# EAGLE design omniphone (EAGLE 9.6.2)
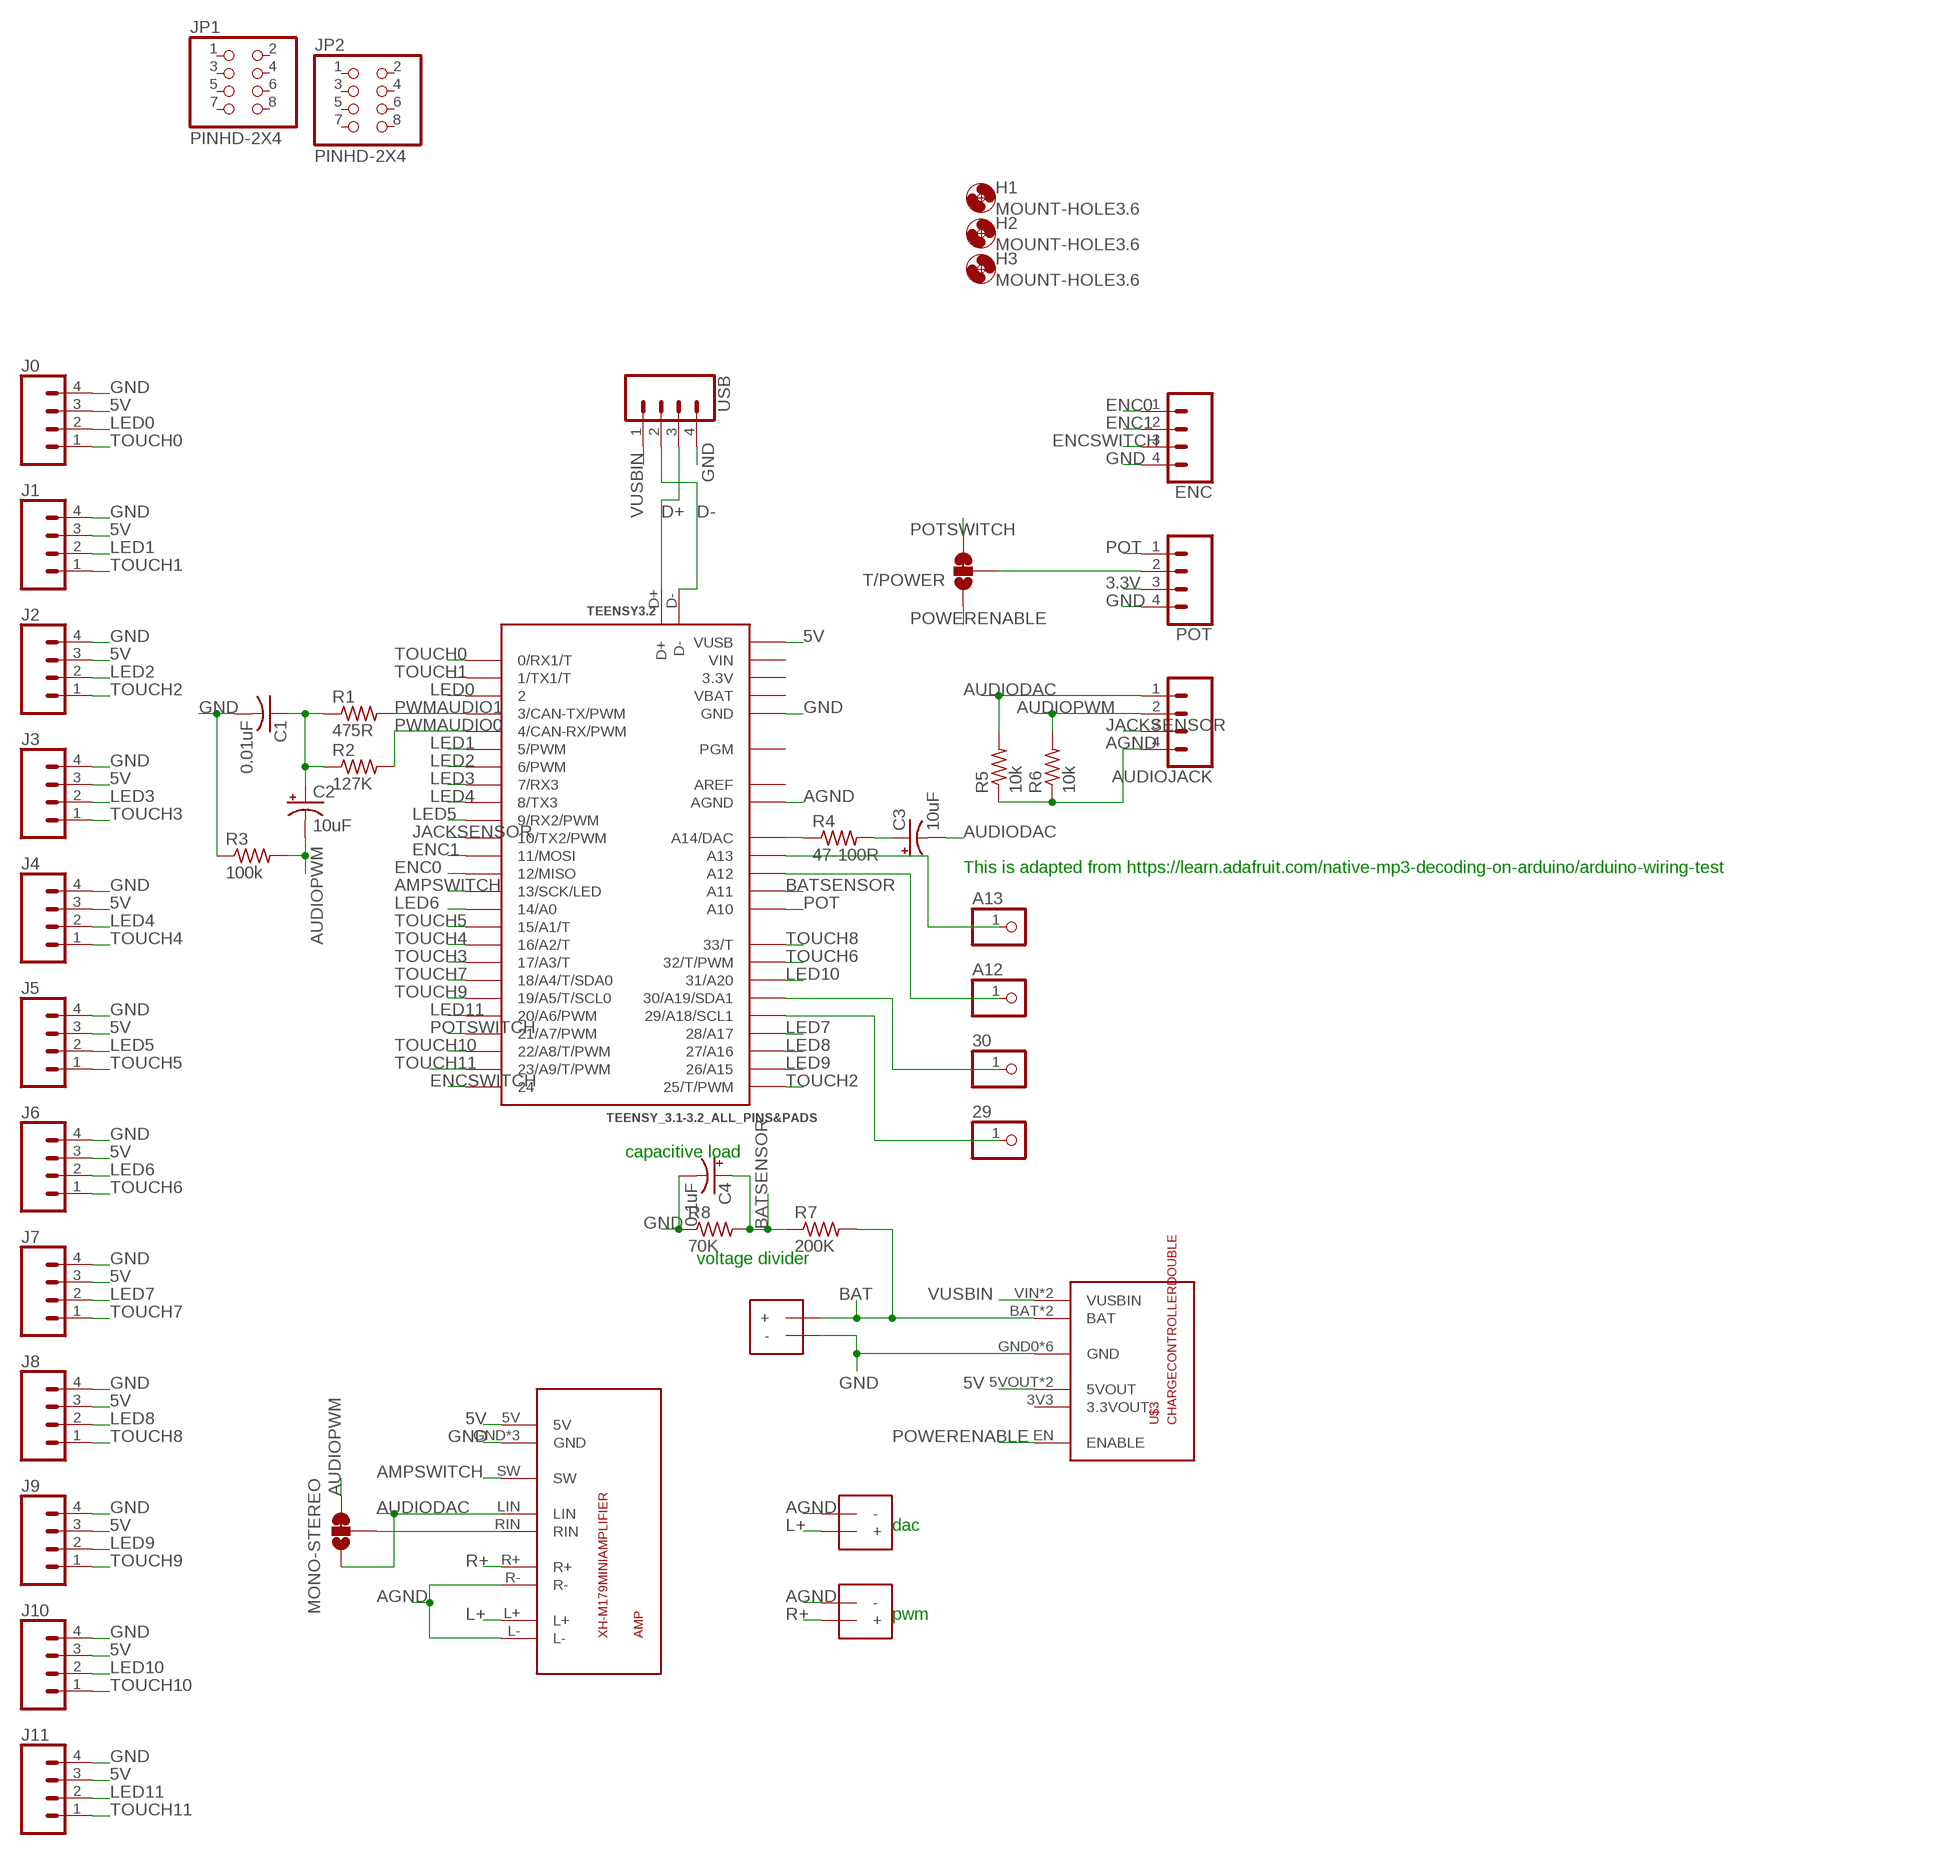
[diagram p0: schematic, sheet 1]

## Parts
29  PINHD-1X1  [1X01]
30  PINHD-1X1  [1X01]
A12  PINHD-1X1  [1X01]
A13  PINHD-1X1  [1X01]
AMP  XH-M179MINIAMPLIFIER  [XH-M179AMP]
AUDIOJACK  CONN_04POLAR_LOCK  [MOLEX-1X4_LOCK]
BATTERY  SPEAKERTERMINAL-3.5MM  [1X2-3.5MM]
C1  0.01uF  C-US025-024X044  [C025-024X044]
C2  10uF  CPOL-USE2-4  [E2-4]
C3  10uF  CPOL-USE2-4  [E2-4]
C4  0.1uF  CPOL-USE2-4  [E2-4]
ENC  CONN_04POLAR_LOCK  [MOLEX-1X4_LOCK]
H1  MOUNT-HOLE3.6  [3,6]
H2  MOUNT-HOLE3.6  [3,6]
H3  MOUNT-HOLE3.6  [3,6]
J0  CONN_04POLAR_LOCK  [MOLEX-1X4_LOCK]
J1  CONN_04POLAR_LOCK  [MOLEX-1X4_LOCK]
J2  CONN_04POLAR_LOCK  [MOLEX-1X4_LOCK]
J3  CONN_04POLAR_LOCK  [MOLEX-1X4_LOCK]
J4  CONN_04POLAR_LOCK  [MOLEX-1X4_LOCK]
J5  CONN_04POLAR_LOCK  [MOLEX-1X4_LOCK]
J6  CONN_04POLAR_LOCK  [MOLEX-1X4_LOCK]
J7  CONN_04POLAR_LOCK  [MOLEX-1X4_LOCK]
J8  CONN_04POLAR_LOCK  [MOLEX-1X4_LOCK]
J9  CONN_04POLAR_LOCK  [MOLEX-1X4_LOCK]
J10  CONN_04POLAR_LOCK  [MOLEX-1X4_LOCK]
J11  CONN_04POLAR_LOCK  [MOLEX-1X4_LOCK]
JP1  PINHD-2X4  [2X04]
JP2  PINHD-2X4  [2X04]
MONO-STEREO  JUMPER-SMT_3_1-NC_TRACE_SILK  [SMT-JUMPER_3_1-NC_TRACE_SILK]
POT  CONN_04POLAR_LOCK  [MOLEX-1X4_LOCK]
R1  475R  R-US_0204/2V  [0204V]
R2  127K  R-US_0204/2V  [0204V]
R3  100k  R-US_0204/2V  [0204V]
R4  47-100R  R-US_0204/2V  [0204V]
R5  10k  R-US_0204/2V  [0204V]
R6  10k  R-US_0204/2V  [0204V]
R7  200K  R-US_0204/2V  [0204V]
R8  70K  R-US_0204/2V  [0204V]
SPEAKERDAC  SPEAKERTERMINAL-3.5MM  [1X2-3.5MM]
SPEAKERPWM  SPEAKERTERMINAL-3.5MM  [1X2-3.5MM]
T/POWER  JUMPER-SMT_3_1-NC_TRACE_SILK  [SMT-JUMPER_3_1-NC_TRACE_SILK]
TEENSY3.2  TEENSY_3.1-3.2_ALL_PINS&PADS  [TEENSY_3.0-3.2_ALL_PINS_&_PADS]
U$3  CHARGECONTROLLERDOUBLE  [CHARGECONTROLLERDOUBLE]
USB  CONN_04POLAR_LOCK  [MOLEX-1X4_LOCK]

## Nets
3.3V: POT.3
5V: AMP.5V J0.3 J1.3 J2.3 J3.3 J4.3 J5.3 J6.3 J7.3 J8.3 J9.3 J10.3 J11.3 TEENSY3.2.VUSB TEENSY3.2.VUSB1(VUSB) U$3.5VOUT U$3.5VOUT1(5VOUT)
AGND: AMP.L- AMP.R- AUDIOJACK.4 R5.1 R6.1 SPEAKERDAC.- SPEAKERPWM.- TEENSY3.2.AGND
AMPSWITCH: AMP.SW TEENSY3.2.13(13/SCK/LED)
AUDIODAC: AMP.LIN AUDIOJACK.1 C3.- MONO-STEREO.1 R5.2
AUDIOPWM: AUDIOJACK.2 C2.- MONO-STEREO.3 R3.2 R6.2
BAT: BATTERY.+ R7.2 U$3.BAT U$3.BAT1(BAT)
BATSENSOR: C4.+ R7.1 R8.2 TEENSY3.2.A11
D+: TEENSY3.2.D+ USB.3
D-: TEENSY3.2.D- USB.2
ENC0: ENC.1 TEENSY3.2.12(12/MISO)
ENC1: ENC.2 TEENSY3.2.11(11/MOSI)
ENCSWITCH: ENC.3 TEENSY3.2.24
GND: AMP.GND AMP.GND1(GND) AMP.GND2(GND) BATTERY.- C1.2 C4.- ENC.4 J0.4 J1.4 J2.4 J3.4 J4.4 J5.4 J6.4 J7.4 J8.4 J9.4 J10.4 J11.4 POT.4 R3.1 R8.1 TEENSY3.2.GND TEENSY3.2.GND1(GND) TEENSY3.2.GND2(GND) TEENSY3.2.GND3(GND) U$3.GND0(GND) U$3.GND1(GND) U$3.GND2(GND) U$3.GND3(GND) U$3.GND4(GND) U$3.GND5(GND) USB.4
JACKSENSOR: AUDIOJACK.3 TEENSY3.2.10(10/TX2/PWM)
L+: AMP.L+ SPEAKERDAC.+
LED0: J0.2 TEENSY3.2.2
LED1: J1.2 TEENSY3.2.5(5/PWM)
LED2: J2.2 TEENSY3.2.6(6/PWM)
LED3: J3.2 TEENSY3.2.7(7/RX3)
LED4: J4.2 TEENSY3.2.8(8/TX3)
LED5: J5.2 TEENSY3.2.9(9/RX2/PWM)
LED6: J6.2 TEENSY3.2.14/A0
LED7: J7.2 TEENSY3.2.28(28/A17)
LED8: J8.2 TEENSY3.2.27(27/A16)
LED9: J9.2 TEENSY3.2.26(26/A15)
LED10: J10.2 TEENSY3.2.31(31/A20)
LED11: J11.2 TEENSY3.2.20/A6(20/A6/PWM)
N$1: C1.1 C2.+ R1.1 R2.1
N$2: A13.1 TEENSY3.2.A13
N$3: A12.1 TEENSY3.2.A12
N$4: POT.2 T/POWER.2
N$5: R4.1 TEENSY3.2.RESET/DAC(A14/DAC)
N$6: 30.1 TEENSY3.2.30(30/A19/SDA1)
N$7: C3.+ R4.2
N$8: 29.1 TEENSY3.2.29(29/A18/SCL1)
POT: POT.1 TEENSY3.2.A10
POTSWITCH: T/POWER.3 TEENSY3.2.21/A7(21/A7/PWM)
POWERENABLE: T/POWER.1 U$3.EN(ENABLE)
PWMAUDIO0: R2.2 TEENSY3.2.4(4/CAN-RX/PWM)
PWMAUDIO1: R1.2 TEENSY3.2.3(3/CAN-TX/PWM)
R+: AMP.R+ SPEAKERPWM.+
RIN: AMP.RIN MONO-STEREO.2
TOUCH0: J0.1 TEENSY3.2.0(0/RX1/T)
TOUCH1: J1.1 TEENSY3.2.1(1/TX1/T)
TOUCH2: J2.1 TEENSY3.2.25(25/T/PWM)
TOUCH3: J3.1 TEENSY3.2.17/A3(17/A3/T)
TOUCH4: J4.1 TEENSY3.2.16/A2(16/A2/T)
TOUCH5: J5.1 TEENSY3.2.15/A1(15/A1/T)
TOUCH6: J6.1 TEENSY3.2.32(32/T/PWM)
TOUCH7: J7.1 TEENSY3.2.18/A4(18/A4/T/SDA0)
TOUCH8: J8.1 TEENSY3.2.33(33/T)
TOUCH9: J9.1 TEENSY3.2.19/A5(19/A5/T/SCL0)
TOUCH10: J10.1 TEENSY3.2.22/A8(22/A8/T/PWM)
TOUCH11: J11.1 TEENSY3.2.23/A9(23/A9/T/PWM)
VUSBIN: U$3.VIN1(VUSBIN) U$3.VIN(VUSBIN) USB.1
Unconnected: JP1.1 JP1.2 JP1.3 JP1.4 JP1.5 JP1.6 JP1.7 JP1.8 JP2.1 JP2.2 JP2.3 JP2.4 JP2.5 JP2.6 JP2.7 JP2.8 TEENSY3.2.PGM U$3.3V3(3.3VOUT)

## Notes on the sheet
- This is adapted from https://learn.adafruit.com/native-mp3-decoding-on-arduino/arduino-wiring-test
- capacitive load
- voltage divider
- dac
- pwm

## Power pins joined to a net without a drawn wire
3.3V: TEENSY3.2.3.3V TEENSY3.2.3.3V1(3.3V) TEENSY3.2.3.3V2(3.3V)
AREF: TEENSY3.2.AREF
VBAT: TEENSY3.2.VBAT
VIN: TEENSY3.2.VIN

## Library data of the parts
29 30 A12 A13 = adafruit:PINHD-1X1: Pin header 1x1 for 0.1" spacing
AMP = ArvidLibrary:XH-M179MINIAMPLIFIER
AUDIOJACK ENC J0 J1-J11 POT USB = SparkFun-Connectors:CONN_04: Multi connection point. Often used as Generic Header-pin footprint for 0.1 inch spaced/style header connections On any of the 0.1 inch spaced packages, you can populate with these: Break Away Headers - Straight (PRT-00116) Break Away Male Headers - Right Angle (PRT-00553) Female Headers (PRT-00115)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; PROD_ID: CONN-08186; SF_ID: PRT-08231
BATTERY SPEAKERDAC SPEAKERPWM = ArvidLibrary:SPEAKERTERMINAL: 3.5mm Terminal block
C1 = adafruit:C-US: CAPACITOR, American symbol
C2-C4 = adafruit:CPOL-US: POLARIZED CAPACITOR, American symbol
H1-H3 = holes:MOUNT-HOLE: MOUNTING HOLE with drill center marker
JP1 JP2 = Connector:PINHD-2X4: PIN HEADER; CATEGORY: CONNECTOR; SUB-CATEGORY: PIN-HEADER
MONO-STEREO T/POWER = SparkFun-Jumpers:JUMPER-SMT_3_1-NC_TRACE: Normally closed trace jumper (1 of 2 connections) This jumper has a trace between two pads so it's normally closed (NC). The other connection is normally open (NO). Use a razor knife to open the connection. For best results follow the IPC guidelines for cutting traces: Cutout at least 0.063 mm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
R1-R8 = adafruit:R-US_: RESISTOR, American symbol
TEENSY3.2 = ArvidLibrary:TEENSY_3.1-3.2_ALL_PINS&PADS: Footprint for Teensy 3.1 or 3.2 board using all pads and all through-holes. Pads need a 2x7 0.1" SMD header. Arvid edit: added USB data and flipped inner pins for easier assembly
U$3 = ArvidLibrary:CHARGECONTROLLERDOUBLE

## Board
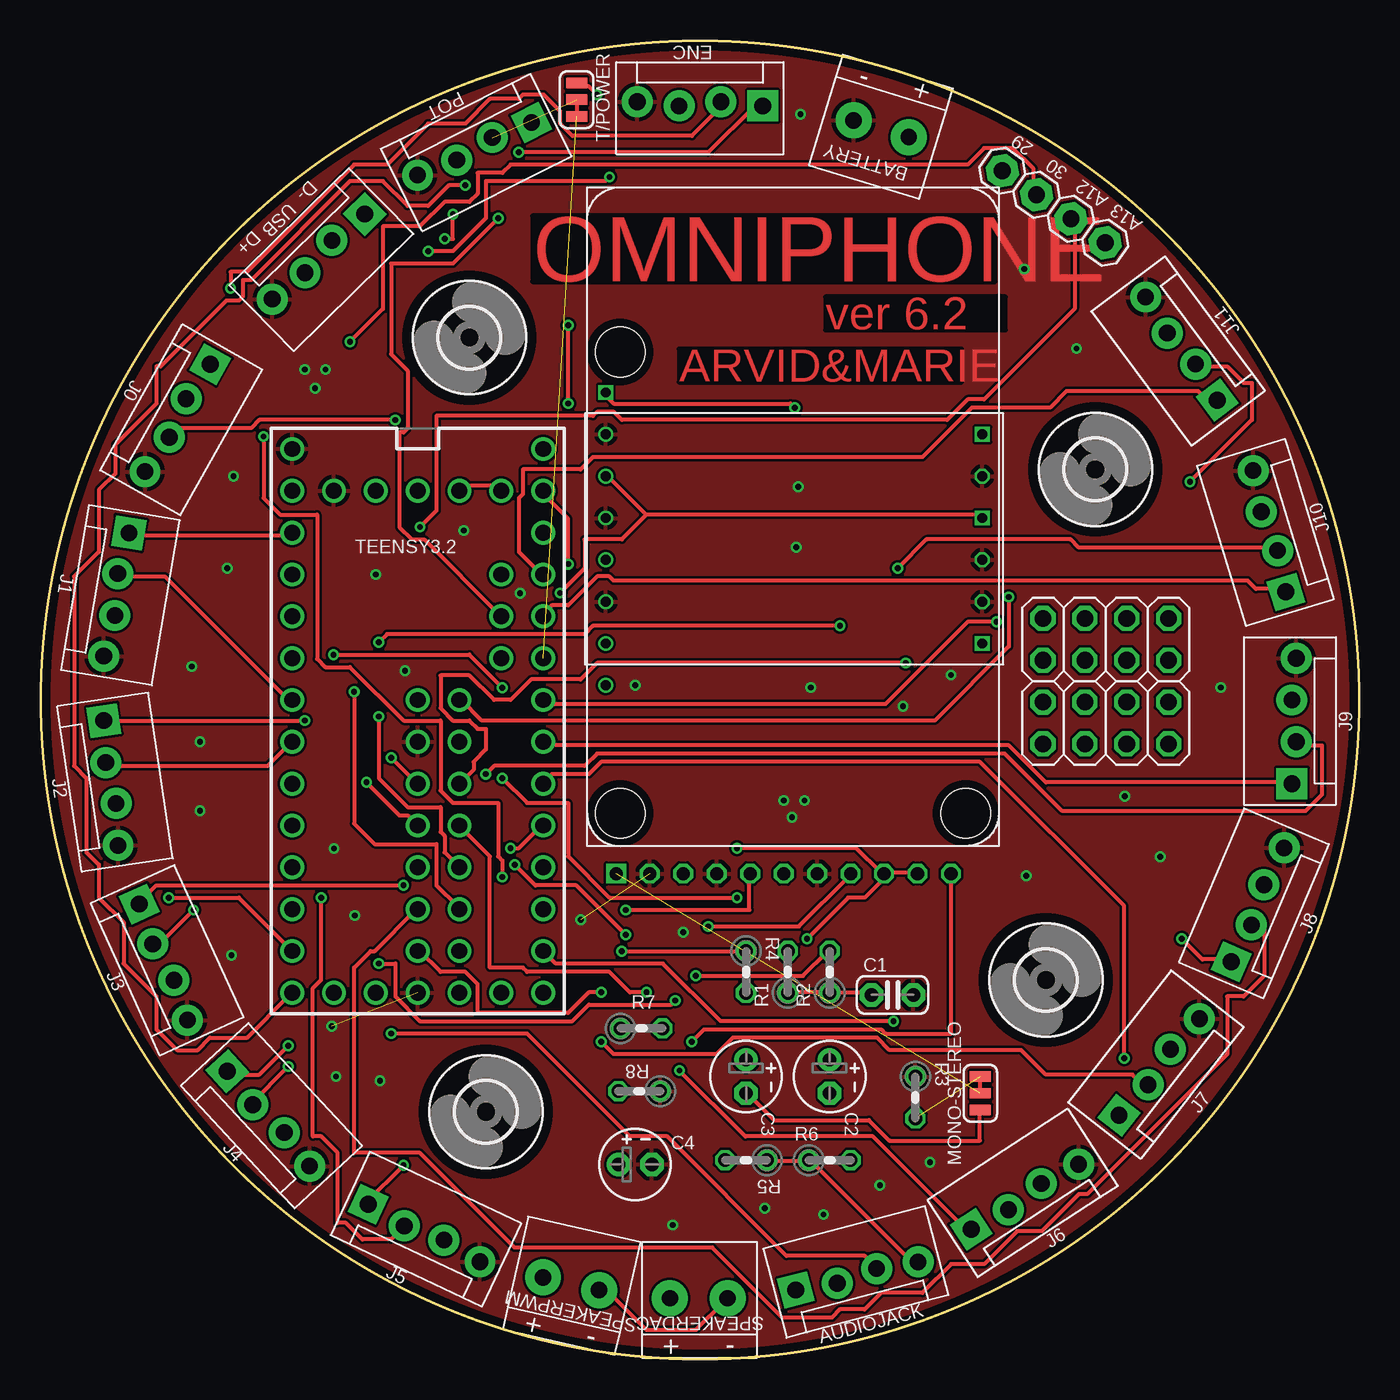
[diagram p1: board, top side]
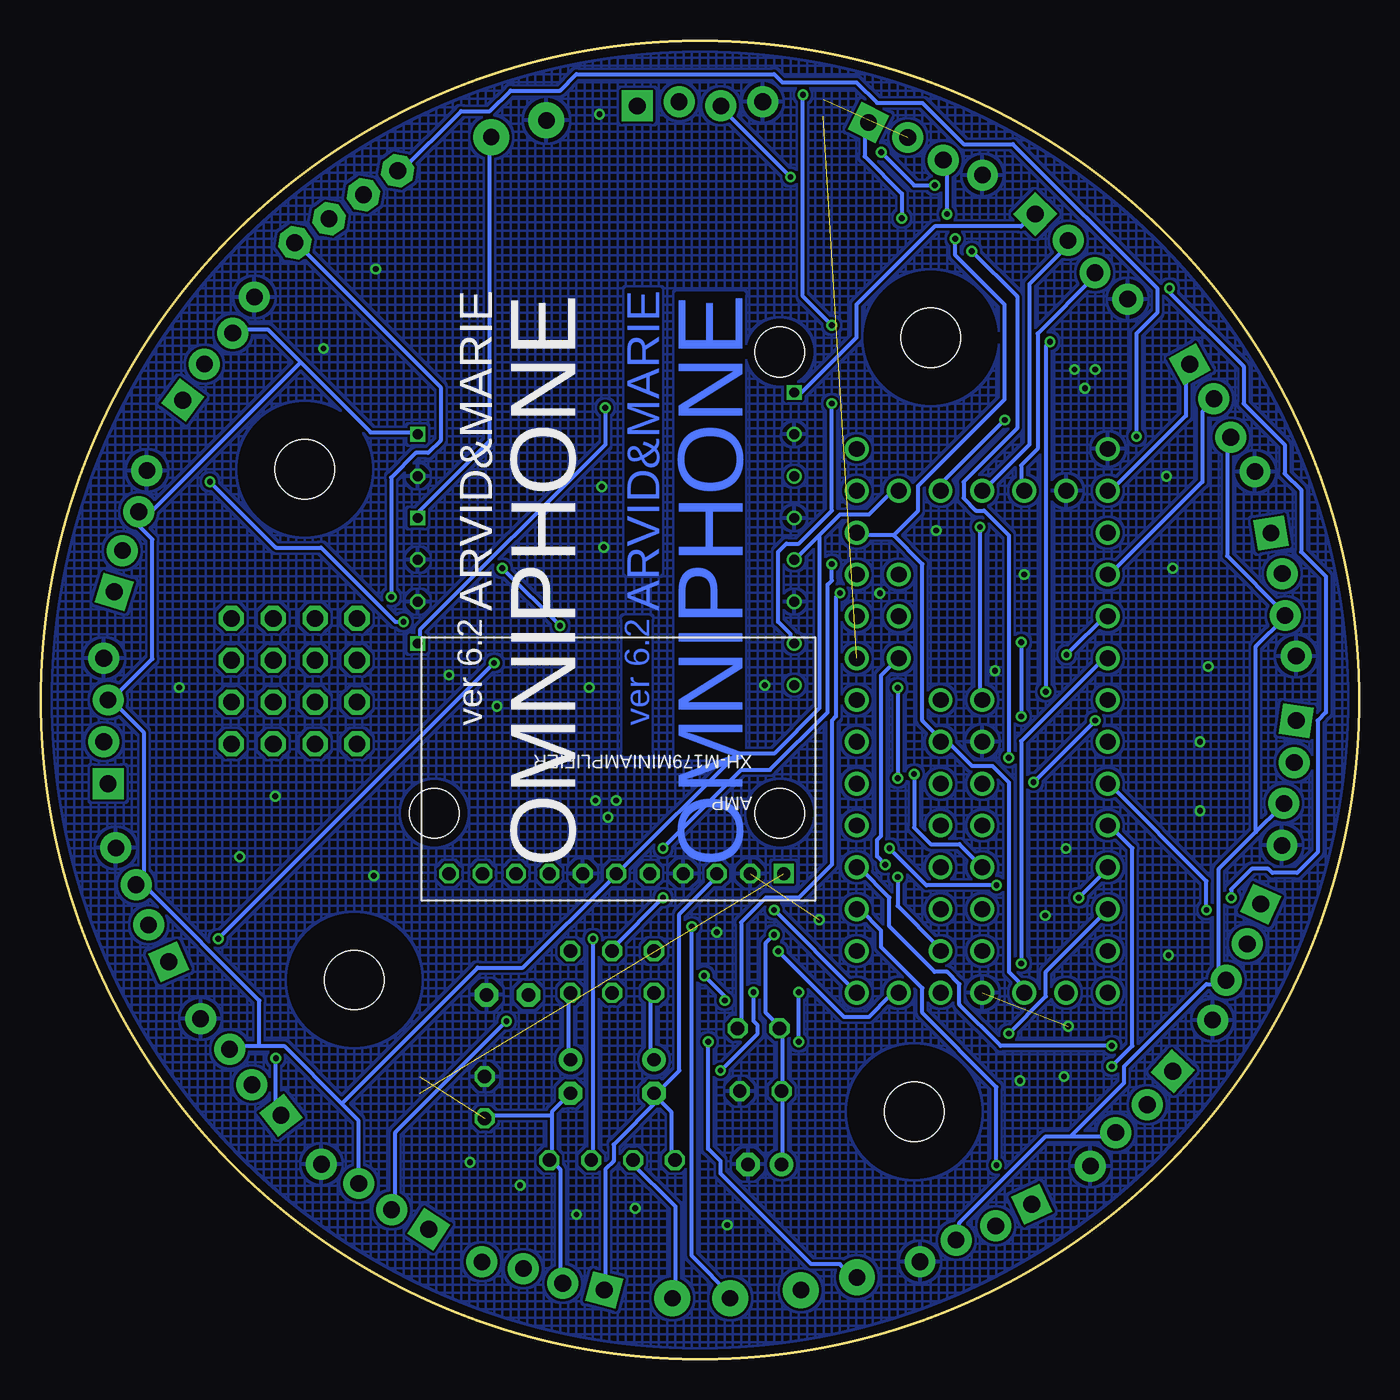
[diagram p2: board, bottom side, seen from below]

Size 80 x 80 mm. Coordinates in mm from the lower left corner, seen from the top.
Outline: circle at 40,40 radius 40
Copper layers (1*16): Top 0.035mm / dielectric 1.6mm / Bottom 0.035mm
Design rules "Elecrow_2-layer_PCB_eagle_rule": minimum track width 6mil, minimum drill 12mil, track to track 6mil, track to pad 6mil, pad to pad 6mil, via to via 8mil, smd to smd 0mil, copper to edge 20mil, drill to drill 10mil, minimum pad ring 6mil, minimum via ring 6mil, stop-mask expansion 0mil, vias tented up to drill 100mil, thermal gap 10mil

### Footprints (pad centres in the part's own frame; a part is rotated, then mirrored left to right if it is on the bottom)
1X01 = drill 1.016 pad 1.93 octagon: 1 0,0
XH-M179AMP = drill 0.8 octagon: 5V 12.065,-1.651; GND 3.937,-1.651; GND1 8.001,-1.651; GND2 14.097,-1.651; L+ 16.129,-1.651; L- 18.161,-1.651; LIN 5.969,-1.651; R+ 22.225,-1.651; R- 20.193,-1.651; SW 10.033,-1.651 | drill 0.8 square: RIN 1.905,-1.651
MOLEX-1X4_LOCK = drill 1.016 pad 1.88 square: 1 0,0.127 | drill 1.016 pad 1.88: 2 2.54,-0.127; 3 5.08,0.127; 4 7.62,-0.127
1X2-3.5MM = drill 1 pad 2.184: + -1.7,0; - 1.8,0
C025-024X044 = drill 0.813 pad 1.422 octagon: 1 -1.27,0; 2 1.27,0
E2-4 = drill 0.813 pad 1.422: + -1.016,0 | drill 0.813 pad 1.422 octagon: - 1.016,0
3,6 = hole 3.6: 0,0
2X04 = drill 1.016 octagon: 1 -3.81,-1.27; 2 -3.81,1.27; 3 -1.27,-1.27; 4 -1.27,1.27; 5 1.27,-1.27; 6 1.27,1.27; 7 3.81,-1.27; 8 3.81,1.27
SMT-JUMPER_3_1-NC_TRACE_SILK = smd 0.635 x 1.27: 1 -1.016,0; 2 0,0; 3 1.016,0
0204V = drill 0.813 octagon: 1 -1.27,0; 2 1.27,0
TEENSY_3.0-3.2_ALL_PINS_&_PADS = drill 0.965: 0 -7.62,13.97; 1 -7.62,11.43; 2 -7.62,8.89; 3 -7.62,6.35; 3.3V 7.62,11.43; 3.3V1 -2.54,-16.51; 3.3V2 2.54,-1.27; 4 -7.62,3.81; 5 -7.62,1.27; 6 -7.62,-1.27; 7 -7.62,-3.81; 8 -7.62,-6.35; 9 -7.62,-8.89; 10 -7.62,-11.43; 11 -7.62,-13.97; 12 -7.62,-16.51; 13 7.62,-16.51; 14/A0 7.62,-13.97; 15/A1 7.62,-11.43; 16/A2 7.62,-8.89; 17/A3 7.62,-6.35; 18/A4 7.62,-3.81; 19/A5 7.62,-1.27; 20/A6 7.62,1.27; 21/A7 7.62,3.81; 22/A8 7.62,6.35; 23/A9 7.62,8.89; 24 0,-3.81; 25 0,-6.35; 26 0,-8.89; 27 0,-11.43; 28 0,-13.97; 29 2.54,-13.97; 30 2.54,-11.43; 31 2.54,-8.89; 32 2.54,-6.35; 33 2.54,-3.81; A10 5.08,6.35; A11 5.08,3.81; A12 0,1.27; A13 2.54,1.27; AGND 7.62,13.97; AREF 5.08,8.89; D+ -2.54,13.97; D- 0,13.97; GND -7.62,16.51; GND1 0,-16.51; GND2 0,-1.27; GND3 -5.08,13.97; PGM 2.54,-16.51; RESET/DAC 5.08,-16.51; VBAT -5.08,-16.51; VIN 7.62,16.51; VUSB 5.08,13.97; VUSB1 2.54,13.97
CHARGECONTROLLERDOUBLE = drill 0.6: 3V3 -22.86,-15.24; 5VOUT1 -22.86,-7.62; BAT1 -22.86,-2.54; EN -22.86,-12.7; GND3 -22.86,0; GND4 -22.86,-5.08; GND5 -22.86,-10.16 | drill 0.6 square: 5VOUT 0,0; BAT 0,-5.08; VIN 0,-12.7; VIN1 -22.86,2.54 | drill 0.6 octagon: GND0 0,-2.54; GND1 0,-7.62; GND2 0,-10.16 | hole 3: -22,-23; -1,-23; -22,5

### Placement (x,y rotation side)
29  58.36,72.13 145 top
30  60.44,70.67 145 top
A12  62.52,69.22 145 top
A13  64.6,67.76 145 top
AMP  33.02,27.81 180 bottom
AUDIOJACK  45.84,4.06 14.8 top
BATTERY  51.05,74.67 163 top
C1  51.68,22.09 0 top
C2  47.87,17.14 270 top
C3  42.79,17.14 270 top
C4  36.06,11.81 0 top
ENC  43.81,76.19 180 top
H1  27,15 0 top
H2  61,23 0 top
H3  64,54 0 top
H4  MOUNT-HOLE3.6  [3,6]  26,62 0 top
J0  10.16,60.45 240.6 top
J1  5.2,50.16 260.4 top
J2  3.68,38.73 278.4 top
J3  5.84,27.55 294.5 top
J4  11.21,17.38 312.8 top
J5  19.81,9.27 334.7 top
J6  56.53,7.76 33.1 top
J7  65.54,14.71 52.1 top
J8  72.37,24.06 67 top
J9  76.07,34.92 90 top
J10  75.69,46.6 107 top
J11  71.5,58.28 126.7 top
JP1  64.64,43.68 0 top
JP2  64.64,38.6 0 top
MONO-STEREO  57.02,16.12 90 top
POT  29.71,75.18 206.7 top
R1  45.33,23.49 90 top
R2  47.87,23.49 90 top
R3  53.08,15.87 270 top
R4  42.79,23.49 270 top
R5  42.79,12.06 180 top
R6  47.87,12.06 0 top
R7  36.44,20.06 0 top
R8  36.32,16.25 180 top
SPEAKERDAC  39.87,3.68 0 top
SPEAKERPWM  32.13,4.57 347.2 top
T/POWER  32.51,76.45 270 top
TEENSY3.2  22.86,38.73 0 top
U$3  57.14,56.13 0 top
USB  19.55,69.59 224.5 top

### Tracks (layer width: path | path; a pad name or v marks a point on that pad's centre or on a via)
3.3V  (via drill 0.35)
  Top 0.254: v25,69.5 25,68 v24.5,68
  Bottom 0.254: TEENSY3.2.3.3V1 20.5,22.25 20.5,22.75 21.25,23.5 21.25,35 22.25,36 23.5,36 24.75,37.25 25.25,37.25 TEENSY3.2.3.3V2 25.25,37.5 26.5,38.75 26.5,48.25 28.25,50 | 28.25,50 30.25,50 TEENSY3.2.3.3V | v25,69.5 25,72.75 POT.3 | v24.5,68 24.5,67 21.5,64 21.5,58.25 26.75,53 26.75,51.5 28.25,50
5V  (via drill 0.35)
  Top 0.254: TEENSY3.2.VUSB1 25.5,52.75 25.75,53 27.5,53 27.75,52.75 TEENSY3.2.VUSB | v21.5,57 13.25,57 12.75,56.5 8.5,56.5 8,56 J0.3
  Bottom 0.254: J0.3 8,55.75 8,48.75 4.5,45.25 J1.3 4.5,45 6.25,43.25 6.25,32 | 17.5,13.5 19,13.5 24.25,8.25 24.25,7.25 J5.3 | 17.5,13.5 15,13.5 J4.3 | 8.5,22.75 9.25,22.75 14.25,17.75 14.25,16.75 17.5,13.5 | 8.5,22.75 8.25,22.75 J3.3 8.5,22.75 | 6.25,32 8.5,29.75 8.5,22.75 | 6.25,32 4.75,33.5 J2.3 | 32.75,50 31.5,51.25 29.75,51.25 28.5,52.5 28,52.5 TEENSY3.2.VUSB | 32.75,50 34,48.75 34.25,48.75 U$3.5VOUT1 | 32.75,50 32.75,39.5 35.5,36.75 37.75,36.75 45,29.5 AMP.5V 45.25,29.25 50.75,23.75 53.5,23.75 61.75,15.5 | 64.25,60.5 66.25,62.5 68.25,62.5 J11.3 | 64.25,60.5 60,56.25 57.25,56.25 U$3.5VOUT | 64.25,60.5 73.25,51.5 74,51.5 J10.3 74,51.25 74,50.5 73.25,49.75 73.25,42.5 75.75,40 | 61.75,15.5 65.25,19 66.75,19 | 61.75,15.5 60.75,14.5 60.75,10.75 J6.3 | 66.75,19 68.5,19 J7.3 | 73.75,28.75 74,28.75 J8.3 73.75,28.75 | 73.75,28.75 66.75,21.75 66.75,19 | 75.75,40 73.75,38 73.75,28.75 | 75.75,40 J9.3 | v21.5,57 25.25,53.25 25.25,52.75 TEENSY3.2.VUSB1
AGND  (via drill 0.35)
  Top 0.254: SPEAKERDAC.- 41.5,3.5 39.75,1.75 36.75,1.75 34.5,4 34,4 SPEAKERPWM.- | R5.1 44.25,12 46.5,12 R6.1 46.75,12 52.75,6 53,6 AUDIOJACK.4 | AMP.L- 51.25,29.5 53,29.5 AMP.R- | v32,48.25 32,51 30.5,52.5 TEENSY3.2.AGND | v42.25,31 49.5,31 51,29.5 AMP.L- | v46.5,25.5 49,28 50,28 51.25,29.25 AMP.L-
  Bottom 0.254: SPEAKERDAC.- 41.5,3.75 41.5,9.25 44.25,12 R5.1 | v32,48.25 32,47.25 32.25,47 32.25,39.25 35.75,35.75 37.5,35.75 v42.25,31 | v46.5,25.5 46.5,12.25 R6.1
AMPSWITCH  (via drill 0.35)
  Top 0.254: v35.5,27.25 43,27.25 43,29.25 AMP.SW
  Bottom 0.254: v35.5,27.25 30.5,22.25 TEENSY3.2.13
AUDIODAC
  Top 0.254: MONO-STEREO.1 57,15 57,13.25 51.5,13.25 50.25,14.5 44.5,14.5 43,16 C3.-
  Bottom 0.254: 42.75,16 41.25,17.5 41.25,27 39,29.25 AMP.LIN | 42.75,16 42.5,15.75 | 42.5,15.75 41.75,15 41.75,12.25 R5.2 | 42.75,16 C3.- 42.5,15.75 | 42.5,15.75 45.25,13 45.25,12 45.75,11.5 45.75,4.25 AUDIOJACK.1
AUDIOPWM  (1 unrouted)
  Bottom 0.254: 49,14.75 49,15 48,16 C2.- | 49,14.75 49,12.25 R6.2 49,12 48.5,11.5 48.5,4.75 AUDIOJACK.2 | 49,14.75 53,14.75 R3.2
BAT  (via drill 0.35)
  Top 0.254: 36.75,51.25 34.5,53.5 U$3.BAT1 | 36.75,51.25 57,51.25 U$3.BAT | v31.5,46.5 33,48 33,49.75 35.25,49.75 36.75,51.25
  Bottom 0.254: v31.5,46.5 31.75,46.25 31.75,39 32,38.75 32,30 34,28 36,28 37.5,26.5 37.5,20.25 R7.2 | BATTERY.+ 52.75,74 52.75,55.75 57.25,51.25 U$3.BAT
BATSENSOR  (via drill 0.35)
  Top 0.254: v28.75,30 30,28.75 32.5,28.75 v35.5,25.75
  Bottom 0.254: C4.+ 35,12 35,16.25 R8.2 35,16.5 35,20 R7.1 35.25,20.25 36,21 36,25.25 v35.5,25.75 | v28.75,30 29.25,30.5 29.25,31.5 29,31.75 29,41.5 28,42.5 TEENSY3.2.A11
D+
  Bottom 0.254: TEENSY3.2.D+ 20.5,52.75 20.5,54.25 19.5,55.25 19.5,62.25 16,65.75 USB.3
D-
  Bottom 0.254: TEENSY3.2.D- 22.75,52.75 20,55.5 20,65.25 17.5,67.75 USB.2
ENC0  (via drill 0.35)
  Top 0.254: v25.75,71.25 24.75,71.25 23.5,70 22.25,70 20.75,71.5 18.75,71.5 12.75,65.5 12.25,65.5 12.25,64.5 12,64.25 11.25,64.25 7.25,60.25 7,60.25 7,58 4.5,55.5 4.5,53.75 3.5,52.75 3.5,49 2,47.5 2,36 2.75,35.25 2.75,30.75 3.5,30 3.5,28 5,26.5 5,24 7,22 7,20 8.25,18.75 9.5,18.75 10.25,19.5 12.5,19.5 15,22 TEENSY3.2.12 | v29,73.25 40.5,73.25 43.25,76 43.75,76 ENC.1
  Bottom 0.254: v25.75,71.25 27,71.25 v29,73.25
ENC1  (via drill 0.35)
  Top 0.254: v7.75,28 12,28 15,25 TEENSY3.2.11 | v11.5,65 11.5,66 12.5,66 19,72.5 21,72.5 23.5,75 25.75,75 27.25,76.5 29,76.5 29.25,76.75 30.5,76.75 31.5,75.75 31.5,75 32.25,74.25 39.5,74.25 41.5,76.25 ENC.2
  Bottom 0.254: v7.75,28 7.75,28.5 6.5,29.75 5.5,29.75 5.25,29.5 3.75,29.5 2.5,30.75 2.5,38.75 2,39.25 2,47.5 3.5,49 3.5,52.75 4.5,53.75 4.5,55.5 7,58 7,60.25 11.5,64.75 v11.5,65
ENCSWITCH  (via drill 0.35)
  Top 0.254: v21.25,36.5 22.75,35 TEENSY3.2.24 | v23.5,67.25 25,67.25 27,69.25 27,71.5 34.25,71.5 v34.5,71.75
  Bottom 0.254: v21.25,36.5 21.25,50 22.75,51.5 23.25,51.5 24,52.25 24,53.25 20.75,56.5 20.75,64.5 v23.5,67.25 | v34.5,71.75 38.75,76 ENC.3
GND  (via drill 0.35)  (2 unrouted)
  other vias: 16.63,58.92 16,60.07 17.27,60.07 20.32,47.62 25.65,50.29 29.08,46.48 36.06,40.89 46.73,40.76 45.08,33.9 46.35,33.9 45.59,32.89 65.78,34.16 67.94,30.48 59.81,29.33 71.62,40.76 17.9,17.14 20.57,16.89 17.65,20.19 19.05,26.92 17.77,30.98 9.65,33.27 11.55,24.51 38.98,25.9 32.76,26.66 22.09,41.78 9.65,37.46 9.14,42.03 11.3,48 11.68,53.59 46.1,75.56 59.69,66.16 62.86,61.34 45.97,52.95 45.84,49.27 55.24,41.52 52.32,39.62 53.97,11.93 50.92,10.54 47.49,8.76 43.94,9.14 38.35,8.12
  pour Top: 40,83.18 60.32,83.18 83.18,60.32 83.18,22.22 57.78,-3.18 22.22,-3.18 -5.72,24.76 -5.72,57.78 17.14,80.64 19.68,83.18
  pour Bottom (hatched): 40,83.18 19.68,83.18 -3.18,60.32 -3.18,22.22 22.22,-3.18 57.78,-3.18 85.72,24.76 85.72,57.78 62.86,80.64 60.32,83.18
JACKSENSOR  (via drill 0.35)
  Top 0.254: v21.25,19.75 29.5,19.75 35.75,13.5 38,13.5 45.25,6.25 50,6.25 50.75,5.5 AUDIOJACK.3
  Bottom 0.254: v21.25,19.75 19,22 19,23.5 15.25,27.25 TEENSY3.2.10
L+  (via drill 0.35)
  Top 0.254: v40.5,26.25 46,26.25 49,29.25 AMP.L+
  Bottom 0.254: v40.5,26.25 40.5,6.25 38,3.75 SPEAKERDAC.+
LED0
  Bottom 0.254: TEENSY3.2.2 15,47.75 9.5,53.25 9.5,57.5 8.75,58.25 J0.2
LED1
  Top 0.254: TEENSY3.2.5 15,40 7.5,47.5 4.75,47.5 J1.2
LED2
  Top 0.254: TEENSY3.2.6 15,37.25 13.75,36 4,36 J2.2
LED3  (via drill 0.35)
  Top 0.254: v9.25,27.25 7.25,25.25 7,25.25 J3.2
  Bottom 0.254: v9.25,27.25 9.25,29 15,34.75 TEENSY3.2.7
LED4  (via drill 0.35)
  Top 0.254: v15,17.75 12.75,15.5 J4.2
  Bottom 0.254: v15,17.75 13.75,19 13.75,31 15,32.25 TEENSY3.2.8
LED5  (via drill 0.35)
  Top 0.254: v17,28 17,23 16.5,22.5 16.5,13.5 17,13.5 18,12.5 18,8.25 18.5,8.25 19.5,7.25 21.25,7.25 22,8 J5.2
  Bottom 0.254: v17,28 15.25,29.75 TEENSY3.2.9
LED6  (via drill 0.35)
  Top 0.254: v51.75,20.5 41.25,20.5 37.75,24 31.25,24 30.5,24.75 TEENSY3.2.14/A0
  Bottom 0.254: v51.75,20.5 58.5,13.75 58.5,9.25 J6.2
LED7  (via drill 0.35)
  Top 0.254: v34,22.25 33.25,22.25 32,21 26.5,21 26.5,22.75 25.75,23.5 24.25,23.5 23,24.75 TEENSY3.2.28 | v34,19.25 34.75,18.5 41,18.5 42,19.5 50.75,19.5 51.5,18.75 59.5,18.75 61,17.25 66.25,17.25 66.75,16.75 67,16.75 J7.2
  Bottom 0.254: v34,19.25 v34,22.25
LED8
  Top 0.254: TEENSY3.2.27 22.75,27.25 20.25,24.75 20,24.75 19,23.75 19,12.5 23,12.5 28.75,6.75 40.75,6.75 45,2.5 48,2.5 48.5,3 50,3 51,4 53.5,4 55.25,5.75 57.25,5.75 59.25,7.75 60.75,7.75 63,10 63.5,10 72,18.5 72,22 73,22 74.25,23.25 74.25,26.25 73.5,26.25 J8.2
LED9  (via drill 0.35)
  Top 0.254: v27,35.5 27.5,36 33,36 33.75,36.75 58.5,36.75 62,33.25 76.75,33.25 77.75,34.25 77.75,37.25 76.25,37.25 J9.2
  Bottom 0.254: v27,35.5 27,32.25 26,31.25 24.25,31.25 23,30 TEENSY3.2.26
LED10  (via drill 0.35)
  Top 0.254: v20.5,39 20.5,35.25 22.25,33.5 24.25,33.5 24.25,32 24.5,31.75 24.5,30.75 25.25,30 TEENSY3.2.31 | v20.5,43.5 21,44 33,44 33.5,44.5 v48.5,44.5 | v52,48 53.75,49.75 62.5,49.75 63,49.25 75,49.25 J10.2
  Bottom 0.254: v20.5,43.5 v20.5,39 | v52,48 v48.5,44.5
LED11  (via drill 0.35)
  Top 0.254: v58,44.75 56.25,44.75 51.25,39.75 30.75,39.75 30.5,40 TEENSY3.2.20/A6 | v69.75,53.25 73.5,57 73.5,59.25 73,59.25 72,60.25 70.25,60.25 J11.2
  Bottom 0.254: v58,44.75 58.5,44.75 63,49.25 65.75,49.25 v69.75,53.25
N$1
  Top 0.254: R1.1 45.5,22.25 47.75,22.25 R2.1 48,22.25 50.25,22.25 C1.1
  Bottom 0.254: C2.+ 48,18.25 48,22 R2.1
N$2  (via drill 0.35)
  Top 0.254: v58.75,46.25 58.75,43.25 54.25,38.75 26.75,38.75 25.5,40 TEENSY3.2.A13
  Bottom 0.254: v58.75,46.25 58.75,53.5 57.25,55 56.5,55 55.75,55.75 55.75,59 64.5,67.75 A13.1
N$3  (via drill 0.35)
  Top 0.254: v23,50.5 24,51.5 24,57.25 33.5,57.25 33.75,57.5 34.75,57.5 35.25,57 55,57 56.25,58.25 57.25,58.25 62.75,63.75 62.75,69 A12.1
  Bottom 0.254: v23,50.5 23,40 TEENSY3.2.A12
N$4  (1 unrouted)
N$5  (via drill 0.35)
  Top 0.254: v35.25,24.75 42.75,24.75 R4.1
  Bottom 0.254: v35.25,24.75 31.25,20.75 29.75,20.75 28.5,22 28,22 TEENSY3.2.RESET/DAC
N$6  (via drill 0.35)
  Top 0.254: v19,40.5 19,32.5 20.25,31.25 24,31.25 24,28.75 25.25,27.5 TEENSY3.2.30 | v18.75,61.75 20.75,63.75 20.75,68.75 23,68.75 24.5,70.25 26,70.25 26.5,70.75 26.5,72 28,72 28.5,72.5 56.25,72.5 57.25,73.5 59,73.5 60.25,72.25 60.25,70.75 30.1
  Bottom 0.254: v19,40.5 19,61.5 v18.75,61.75
N$7
  Bottom 0.254: R4.2 43,22 43,18.25 C3.+
N$8  (via drill 0.35)
  Top 0.254: v28,29.25 28,30.25 27.75,30.5 27.75,33.75 25,33.75 24.25,34.5 24.25,38.75 22,38.75 18.75,42 17.25,42 16.75,42.5 16.75,51.25 14.5,51.25 13.5,52.25 v13.5,56
  Bottom 0.254: v28,29.25 28,27.5 25.5,25 TEENSY3.2.29 | v13.5,56 13.5,62.25 12.25,63.5 12.25,65 21,73.75 24,73.75 26.5,76.25 29.25,76.25 30.5,77.5 35,77.5 35.5,78 47.5,78 48.5,77 51.5,77 52.75,75.75 54.5,75.75 58.25,72 29.1
POT  (via drill 0.35)
  Top 0.254: v27.75,69.25 25,66.5 21.25,66.5 21.25,61 22.25,60 22.25,56.5 22,56.25 21.75,56.25 21.75,50.5 22.5,49.75 23.25,49.75 27.75,45.25 TEENSY3.2.A10
  Bottom 0.254: v27.75,69.25 27.75,70.75 30,73 30,75 POT.1
POTSWITCH  (1 unrouted)
POWERENABLE  (via drill 0.35)
  Top 0.254: v33.75,76.75 33.25,77.25 32.75,77.25 T/POWER.1 | v32,58 v32,62.75
  Bottom 0.254: v33.75,76.75 33.75,64.5 v32,62.75 | v32,58 32,51.5 34,49.5 34.75,49.5 35.25,49 35.25,44.75 34.5,44 34.5,43.5 U$3.EN
PWMAUDIO0  (via drill 0.35)
  Top 0.254: v39.75,23.25 46.25,23.25 47.75,24.75 R2.2 | v38.5,21.75 38.25,21.5 33.25,21.5 32.25,20.5 23,20.5 21.5,22 21.5,24 v20.5,24
  Bottom 0.254: v39.75,23.25 38.5,22 v38.5,21.75 | v20.5,24 20.5,37.5 15.25,42.75 TEENSY3.2.4
PWMAUDIO1  (via drill 0.35)
  Top 0.254: v42.25,28 34.5,28 32,30.5 32,33.75 29.5,33.75 v28,35.25 | v28,40.75 26,42.75 v17.75,42.75
  Bottom 0.254: v42.25,28 45.25,25 R1.2 | v28,40.75 v28,35.25 | v17.75,42.75 15.25,45.25 TEENSY3.2.3
R+  (via drill 0.35)
  Top 0.254: v39.5,19.25 40.25,20 51,20 51.25,19.75 55.25,19.75 55.25,29.25 AMP.R+
  Bottom 0.254: v39.5,19.25 39.5,12.75 38.75,12 38.75,11.25 33.25,5.75 31.5,5.75 30.5,4.75 SPEAKERPWM.+
RIN  (1 unrouted)
TOUCH0
  Bottom 0.254: TEENSY3.2.0 15,52.75 10.5,57.25 10.5,60.25 J0.1
TOUCH1
  Top 0.254: TEENSY3.2.1 15,50 5.5,50 J1.1
TOUCH2  (via drill 0.35)
  Top 0.254: v19.75,35 21.75,33 22.25,33 22.75,32.5 TEENSY3.2.25 | v16,38.75 4,38.75 J2.1
  Bottom 0.254: v16,38.75 v19.75,35
TOUCH3  (via drill 0.35)
  Top 0.254: v28.5,31 29,31 30.25,32.25 TEENSY3.2.17/A3 | v22,28.75 7,28.75 6,27.75 J3.1
  Bottom 0.254: v28.5,31 26.25,28.75 v22,28.75
TOUCH4  (via drill 0.35)
  Top 0.254: v15,19 13.25,17.25 11.5,17.25 J4.1
  Bottom 0.254: v15,19 21.75,19 24.25,21.5 24.25,22.75 25,23.5 25.75,23.5 28.5,26.25 28.5,28 30.25,29.75 TEENSY3.2.16/A2
TOUCH5  (via drill 0.35)
  Top 0.254: v22,11.75 19.75,9.5 J5.1
  Bottom 0.254: v22,11.75 22,16.5 26.5,21 26.5,22.5 29,25 29,26 30.25,27.25 TEENSY3.2.15/A1
TOUCH6  (via drill 0.35)
  Top 0.254: v36.75,22.25 35.75,22.25 34.5,23.5 29.5,23.5 29.25,23.75 27.25,23.75 27.25,30.5 25.5,32.25 TEENSY3.2.32 | v38.75,17.5 42.75,13.5 50.5,13.5 56,8 56.25,8 J6.1
  Bottom 0.254: v36.75,22.25 36.75,20.5 36.5,20.25 36.5,19.75 v38.75,17.5
TOUCH7  (via drill 0.35)
  Top 0.254: v65.75,18.25 65.75,27.5 57,36.25 34,36.25 33.25,35.5 31,35.5 30.5,35 TEENSY3.2.18/A4
  Bottom 0.254: v65.75,18.25 65.75,15.25 65.5,15 J7.1
TOUCH8  (via drill 0.35)
  Top 0.254: v52.5,42.25 33.75,42.25 32.75,41.25 29.75,41.25 28.5,40 27.5,40 26,41.5 24.25,41.5 24.25,39.5 25,38.75 26,38.75 26.5,38.25 27,38.25 27,37 26.25,36.25 26.25,35.75 25.5,35 TEENSY3.2.33 | v69.25,25.5 70.5,24.25 72.25,24.25 J8.1
  Bottom 0.254: v69.25,25.5 v52.5,42.25
TOUCH9
  Top 0.254: TEENSY3.2.19/A5 30.5,37.25 58.75,37.25 61,35 75.75,35 J9.1
TOUCH10
  Top 0.254: TEENSY3.2.22/A8 30.5,45.25 31,45.75 32,45.75 33.75,47.5 34.5,47.5 34.75,47.25 73.25,47.25 73.75,46.75 75.5,46.75 J10.1
TOUCH11
  Top 0.254: TEENSY3.2.23/A9 30.25,47.75 29,49 29,52.25 29.25,52.5 29.25,54 32.75,54 33.5,54.75 53.5,54.75 56.5,57.75 61.25,57.75 62.25,58.75 70.25,58.75 70.75,58.25 71.25,58.25 J11.1
VUSBIN  (via drill 0.35)
  Top 0.254: v45.75,57.75 45.5,58 34.75,58 34.25,58.5 U$3.VIN1
  Bottom 0.254: U$3.VIN1 34.25,58.5 34,58.5 30.5,62 30.5,64 25.75,68.75 20.5,68.75 19.75,69.5 USB.1 | v45.75,57.75 45.75,55.5 57,44.25 57,43.5 U$3.VIN

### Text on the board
Top: OMNIPHONE | ver 6.2 | ARVID&MARIE
Bottom: OMNIPHONE | ARVID&MARIE | ver 6.2
tPlace: D- | D+
bPlace: OMNIPHONE | ARVID&MARIE | ver 6.2

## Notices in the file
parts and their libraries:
SparkFun-Connectors: Licensing: Creative Commons ShareAlike 4.0 International - https://creativecommons.org/licenses/by-sa/4.0
